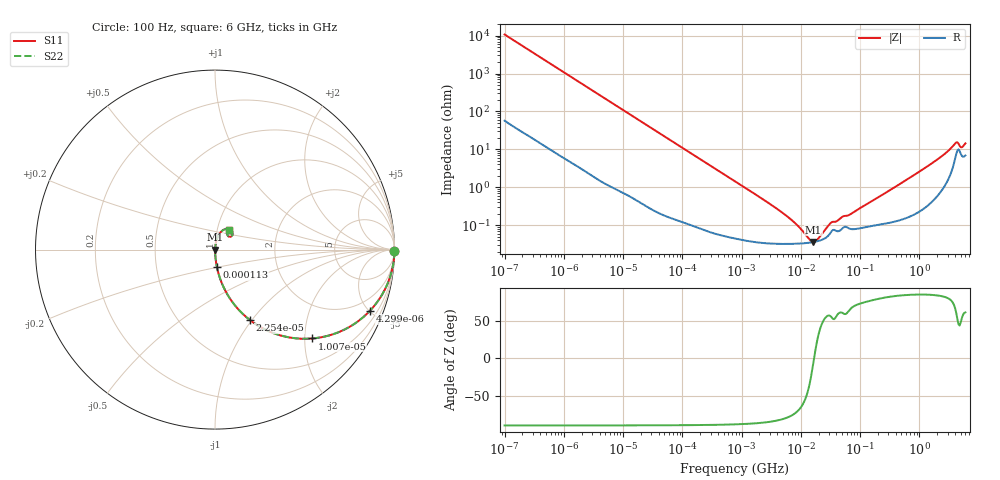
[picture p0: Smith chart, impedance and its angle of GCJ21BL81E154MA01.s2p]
!Murata Part Number: GCJ21BL81E154MA01
!These Parameters are Measured in Series Mode Connection
!Data Generated on Mar 13, 2026
!  o--ll--o
!Port1  Port2
!  o------o
!Operation Temp=25[degC], DC Bias Voltage=0[V]
!Freq. Start=100[Hz] Stop=6[GHz] 401[Steps]
# Hz S RI R 50
!Freq.(Hz) S11(Real) S11(Imag) S21(Real) S21(Imag) S12(Real) S12(Imag) S22(Real) S22(Imag)
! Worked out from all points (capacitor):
!   401 points, 100 Hz to 6 GHz, reference 50 ohm
!   read as one part in series: C = 148 nF near 109 Hz
!   lowest |Z| = 36 mohm at 16.27 MHz (marker M1)
!   series resonance near 16.75 MHz, so ESL is about 610 pH
!   S11 on the Smith chart (normalised r, x): 100 Hz: open; 4.299 kHz: 1.03, -5.06; 10.07 kHz: 1.01, -2.17; 22.54 kHz: 1.01, -0.97; 113 kHz: 1.00, -0.20; 6 GHz: 1.14, +0.25
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100  0.9999 -0.00931  0.000136 0.00931  0.000136 0.00931  0.9999 -0.00931
600  0.9966 -0.0553  0.00336 0.0553  0.00336 0.0553  0.9966 -0.0553
2008  0.966 -0.1786  0.034 0.1786  0.034 0.1786  0.966 -0.1786
4299  0.8635 -0.3405  0.1365 0.3405  0.1365 0.3405  0.8635 -0.3405
6433  0.7402 -0.4356  0.2598 0.4356  0.2598 0.4356  0.7402 -0.4356
10066  0.54 -0.4952  0.46 0.4952  0.46 0.4952  0.54 -0.4952
22537  0.1927 -0.3909  0.8073 0.3909  0.8073 0.3909  0.1927 -0.3909
40335  0.0706 -0.2523  0.9294 0.2523  0.9294 0.2523  0.0706 -0.2523
112960  0.0105 -0.0964  0.9895 0.0964  0.9895 0.0964  0.0105 -0.0964
774597  0.00065 -0.0144  0.9993 0.0144  0.9993 0.0144  0.00065 -0.0144
5554849  0.000323 -0.0018  0.9997 0.0018  0.9997 0.0018  0.000323 -0.0018
8692127  0.000325 -0.000947  0.9997 0.000947  0.9997 0.000947  0.000325 -0.000947
1.555665e7  0.000353 -9.98e-05  0.9996 9.98e-05  0.9996 9.98e-05  0.000353 -9.98e-05
1.626902e7  0.000358 -3.93e-05  0.9996 3.93e-05  0.9996 3.93e-05  0.000358 -3.93e-05
1.946e7  0.00038 0.000205  0.9996 -0.000205  0.9996 -0.000205  0.00038 0.000205
3.330331e7  0.000699 0.000972  0.9993 -0.000972  0.9993 -0.000972  0.000699 0.000972
6.817316e7  0.000801 0.00175  0.9992 -0.00175  0.9992 -0.00175  0.000801 0.00175
3.124326e8  0.00122 0.0081  0.9988 -0.0081  0.9988 -0.0081  0.00122 0.0081
1.791126e9  0.00693 0.0466  0.9931 -0.0466  0.9931 -0.0466  0.00693 0.0466
4.009986e9  0.0667 0.1158  0.9333 -0.1158  0.9333 -0.1158  0.0667 0.1158
5.245841e9  0.0697 0.0801  0.9303 -0.0801  0.9303 -0.0801  0.0697 0.0801
6e9  0.0776 0.1087  0.9224 -0.1087  0.9224 -0.1087  0.0776 0.1087
